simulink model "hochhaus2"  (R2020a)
settings: Solver=ode45  StartTime=0.0  StopTime=5  MaxStep=3e-3  RelTol=1e-3  EnableMultiTasking=on

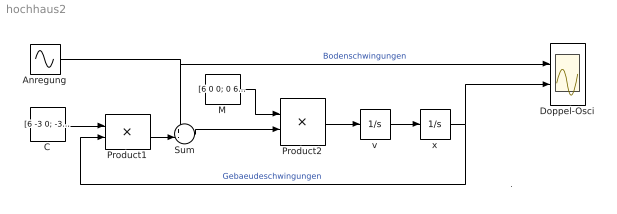
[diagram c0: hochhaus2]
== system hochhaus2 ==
  note: .
  Anregung : Sin  Amplitude=[1; 0; 0]*1e3  Frequency=12  SampleTime=0
  C : Constant  Value=[6 -3 0; -3 4 -1; 0 -1 1]*1e6  VectorParams1D=off
  Doppel-Osci : Scope  NumInputPorts=2
  M : Constant  Value=[6 0 0; 0 6 0; 0 0 1]*1e3  VectorParams1D=off
  Product1 : Product  Multiplication=Matrix(*)  InputSameDT=on  SaturateOnIntegerOverflow=on
  Product2 : Product  Inputs=/*  Multiplication=Matrix(*)  InputSameDT=on  SaturateOnIntegerOverflow=on
  Sum : Sum  Inputs=+-|  InputSameDT=on  SaturateOnIntegerOverflow=on
  v : Integrator  InitialCondition=[0; 0; 0]
  x : Integrator  InitialCondition=[0; 0; 0]
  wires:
  v/1 -> x/1
  Anregung/1 -> Sum/1, Doppel-Osci/1  "Bodenschwingungen"
  x/1 -> Product1/2, Doppel-Osci/2  "Gebaeudeschwingungen"
  Product1/1 -> Sum/2
  C/1 -> Product1/1
  Sum/1 -> Product2/2
  Product2/1 -> v/1
  M/1 -> Product2/1
